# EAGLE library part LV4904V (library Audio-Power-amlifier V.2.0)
SANYO-15W + 15W AUDIO POWER AMPLIFIER
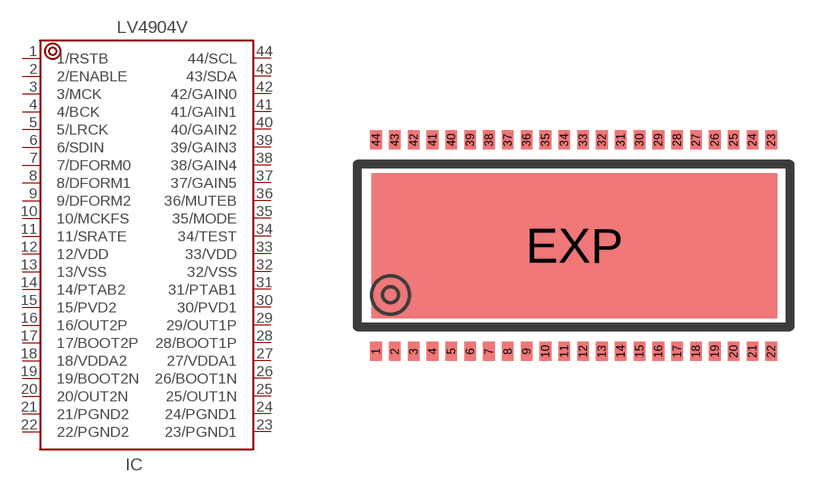
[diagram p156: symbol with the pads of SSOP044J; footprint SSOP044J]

Designator prefix IC

## LV4904V  [SSOP044J]
1  1/RSTB  in
2  2/ENABLE  in
3  3/MCK  in
4  4/BCK  in
5  5/LRCK  in
6  6/SDIN  in
7  7/DFORM0  in
8  8/DFORM1  in
9  9/DFORM2  in
10  10/MCKFS  in
11  11/SRATE  in
12  12/VDD  pwr
13  13/VSS  pwr
14  14/PTAB2
15  15/PVD2
16  16/OUT2P  out
17  17/BOOT2P  out
18  18/VDDA2  pwr
19  19/BOOT2N  out
20  20/OUT2N  out
21  21/PGND2  pwr
22  22/PGND2  pwr
23  23/PGND1  pwr
24  24/PGND1  pwr
25  25/OUT1N  out
26  26/BOOT1N  out
27  27/VDDA1  pwr
28  28/BOOT1P  out
29  29/OUT1P  out
30  30/PVD1
31  31/PTAB1
32  32/VSS  pwr
33  33/VDD  pwr
34  34/TEST  in
35  35/MODE  in
36  36/MUTEB  in
37  37/GAIN5  in
38  38/GAIN4  in
39  39/GAIN3  in
40  40/GAIN2  in
41  41/GAIN1  in
42  42/GAIN0  in
43  43/SDA
44  44/SCL  in

## Footprint SSOP044J (pad centres in mm)
SANYO : SSOP44J(275mil)
smd 0.4 x 0.65: 1 -7.15,-3.65; 2 -6.5,-3.65; 3 -5.85,-3.65; 4 -5.2,-3.65; 5 -4.55,-3.65; 6 -3.9,-3.65; 7 -3.25,-3.65; 8 -2.6,-3.65; 9 -1.95,-3.65; 10 -1.3,-3.65; 11 -0.65,-3.65; 12 0,-3.65; 13 0.65,-3.65; 14 1.3,-3.65; 15 1.95,-3.65; 16 2.6,-3.65; 17 3.25,-3.65; 18 3.9,-3.65; 19 4.55,-3.65; 20 5.2,-3.65; 21 5.85,-3.65; 22 6.5,-3.65; 23 6.5,3.65; 24 5.85,3.65; 25 5.2,3.65; 26 4.55,3.65; 27 3.9,3.65; 28 3.25,3.65; 29 2.6,3.65; 30 1.95,3.65; 31 1.3,3.65; 32 0.65,3.65; 33 0,3.65; 34 -0.65,3.65; 35 -1.3,3.65; 36 -1.95,3.65; 37 -2.6,3.65; 38 -3.25,3.65; 39 -3.9,3.65; 40 -4.55,3.65; 41 -5.2,3.65; 42 -5.85,3.65; 43 -6.5,3.65; 44 -7.15,3.65
smd 14 x 5: EXP -0.3,0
